FUNCTION "GestioneUscite" : VOID
TITLE =Gestione Uscite
//Gestisce le uscite controllando anche che siano rispettate le opportune
//sicurezze
VERSION : 0.1

BEGIN
NETWORK
TITLE =Uilità varie
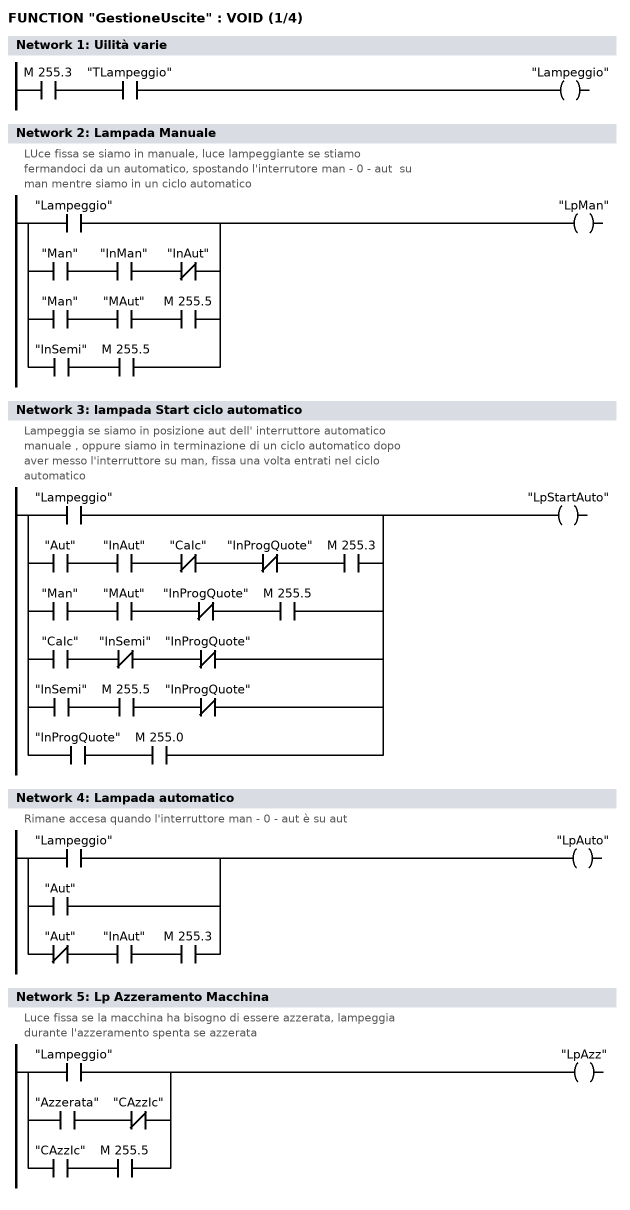
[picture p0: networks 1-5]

      U     M    255.3;
      U     "TLampeggio";
      =     "Lampeggio";


NETWORK
TITLE =Lampada Manuale
//LUce fissa se siamo in manuale, luce lampeggiante se stiamo
//fermandoci da un automatico, spostando l'interrutore man - 0 - aut  su
//man mentre siamo in un ciclo automatico
      O     "Lampeggio";
      O(    ;
      U     "Man";
      U     "InMan";
      UN    "InAut";
      )     ;
      O(    ;
      U     "Man";
      U     "MAut";
      U     M    255.5;
      )     ;
      O(    ;
      U     "InSemi";
      U     M    255.5;
      )     ;
      =     "LpMan";



NETWORK
TITLE =lampada Start ciclo automatico
//Lampeggia se siamo in posizione aut dell' interruttore automatico
//manuale , oppure siamo in terminazione di un ciclo automatico dopo
//aver messo l'interruttore su man, fissa una volta entrati nel ciclo
//automatico
      O     "Lampeggio";
      O(    ;
      U     "Aut";
      U     "InAut";
      UN    "CaIc";
      UN    "InProgQuote";
      U     M    255.3;
      )     ;
      O(    ;
      U     "Man";
      U     "MAut";
      UN    "InProgQuote";
      U     M    255.5;
      )     ;
      O(    ;
      U     "CaIc";
      UN    "InSemi";
      UN    "InProgQuote";
      )     ;
      O(    ;
      U     "InSemi";
      U     M    255.5;
      UN    "InProgQuote";
      )     ;
      O(    ;
      U     "InProgQuote";
      U     M    255.0;
      )     ;
      =     "LpStartAuto";


NETWORK
TITLE =Lampada automatico
//Rimane accesa quando l'interruttore man - 0 - aut è su aut
      O     "Lampeggio";
      O     "Aut";
      O(    ;
      UN    "Aut";
      U     "InAut";
      U     M    255.3;
      )     ;
      =     "LpAuto";


NETWORK
TITLE =Lp Azzeramento Macchina
//Luce fissa se la macchina ha bisogno di essere azzerata, lampeggia
//durante l'azzeramento spenta se azzerata

      O     "Lampeggio";
      O(    ;
      U     "Azzerata";
      UN    "CAzzIc";
      )     ;
      O(    ;
      U     "CAzzIc";
      U     M    255.5;
      )     ;
      =     "LpAzz";

NETWORK
TITLE =Lampada allarmi
//Se la macchina è in allarme, lampeggia
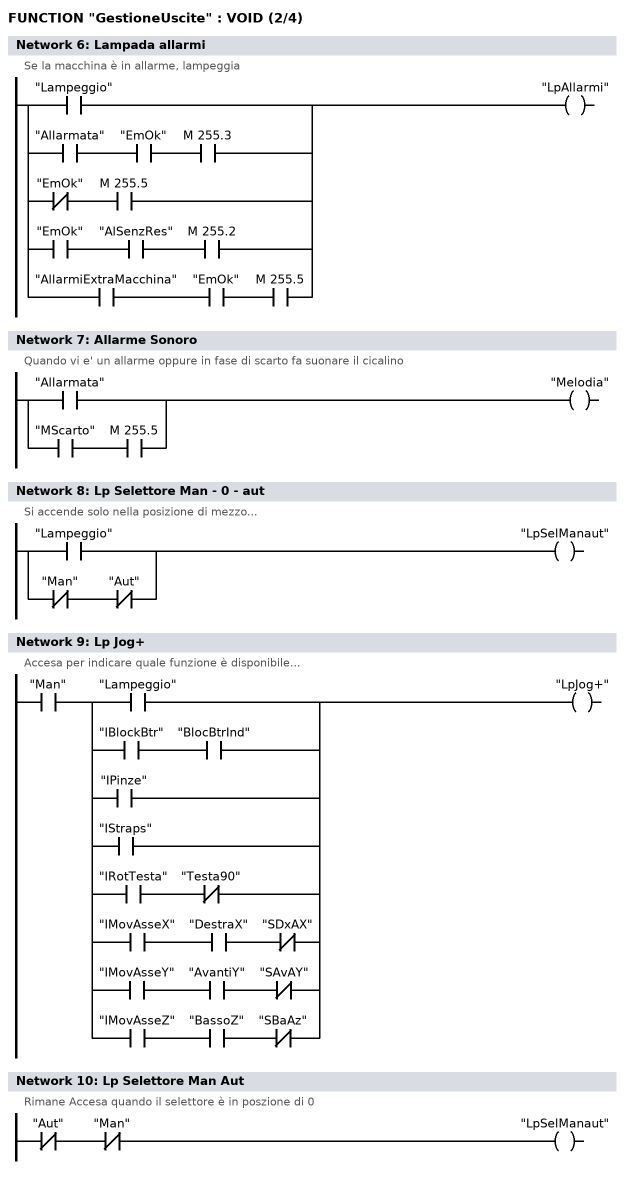
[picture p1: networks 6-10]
      O     "Lampeggio";
      O(    ;
      U     "Allarmata";
      U     "EmOk";
      U     M    255.3;
      )     ;
      O(    ;
      UN    "EmOk";
      U     M    255.5;
      )     ;
      O(    ;
      U     "EmOk";
      U     "AlSenzRes";
      U     M    255.2;
      )     ;
      O(    ;
      U     "AllarmiExtraMacchina";
      U     "EmOk";
      U     M    255.5;
      )     ;
      =     "LpAllarmi";


NETWORK
TITLE =Allarme Sonoro
//Quando vi e' un allarme oppure in fase di scarto fa suonare il cicalino
      O     "Allarmata";
      O(    ;
      U     "MScarto";
      U     M    255.5;
      )     ;
      =     "Melodia";


NETWORK
TITLE =Lp Selettore Man - 0 - aut
//Si accende solo nella posizione di mezzo...
      O     "Lampeggio";
      O(    ;
      UN    "Man";
      UN    "Aut";
      )     ;
      =     "LpSelManaut";

NETWORK
TITLE =Lp Jog+
//Accesa per indicare quale funzione è disponibile...
      U     "Man";
      U(    ;
      O     "Lampeggio";
      O(    ;
      U     "IBlockBtr";
      U     "BlocBtrInd";
      )     ;
      O     "IPinze";
      O     "IStraps";
      O(    ;
      U     "IRotTesta";
      UN    "Testa90";
      )     ;
      O(    ;
      U     "IMovAsseX";
      U     "DestraX";
      UN    "SDxAX";
      )     ;
      O(    ;
      U     "IMovAsseY";
      U     "AvantiY";
      UN    "SAvAY";
      )     ;
      O(    ;
      U     "IMovAsseZ";
      U     "BassoZ";
      UN    "SBaAz";
      )     ;
      )     ;
      =     "LpJog+";


NETWORK
TITLE =Lp Selettore Man Aut
//Rimane Accesa quando il selettore è in poszione di 0
      UN    "Aut";
      UN    "Man";
      =     "LpSelManaut";


NETWORK
TITLE =Motore pompa olio
//Fa Partire la pompa dell'olio
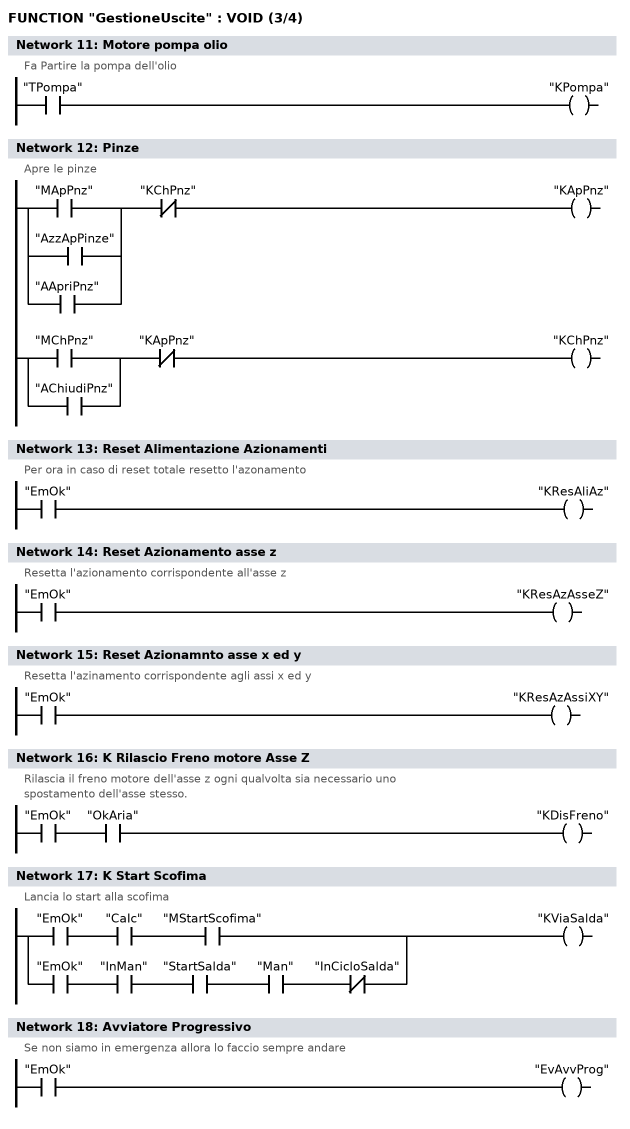
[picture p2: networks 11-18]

      U     "TPompa";
      =     "KPompa";

NETWORK
TITLE =Pinze
//Apre le pinze
      U(    ;
      O     "MApPnz";
      O     "AzzApPinze";
      O     "AApriPnz";
      )     ;
      UN    "KChPnz";
      =     "KApPnz";

      U(    ;
      O     "MChPnz";
      O     "AChiudiPnz";
      )     ;
      UN    "KApPnz";
      =     "KChPnz";


NETWORK
TITLE =Reset Alimentazione Azionamenti
//Per ora in caso di reset totale resetto l'azonamento

      U     "EmOk";
      =     "KResAliAz";

NETWORK
TITLE =Reset Azionamento asse z
//Resetta l'azionamento corrispondente all'asse z
      U     "EmOk";
      =     "KResAzAsseZ";


NETWORK
TITLE =Reset Azionamnto asse x ed y
//Resetta l'azinamento corrispondente agli assi x ed y

      U     "EmOk";
      =     "KResAzAssiXY";

NETWORK
TITLE =K Rilascio Freno motore Asse Z
//Rilascia il freno motore dell'asse z ogni qualvolta sia necessario uno
//spostamento dell'asse stesso.
      U     "EmOk";
      U     "OkAria";
      =     "KDisFreno";


NETWORK
TITLE =K Start Scofima
//Lancia lo start alla scofima
      O(    ;
      U     "EmOk";
      U     "CaIc";
      U     "MStartScofima";
      )     ;
      O(    ;
      U     "EmOk";
      U     "InMan";
      U     "StartSalda";
      U     "Man";
      UN    "InCicloSalda";
      )     ;
      =     "KViaSalda";

NETWORK
TITLE =Avviatore Progressivo
//Se non siamo in emergenza allora lo faccio sempre andare
      U     "EmOk";
      =     "EvAvvProg";


NETWORK
TITLE =Blocco BAtteria
//Manovra il bloccabatteria
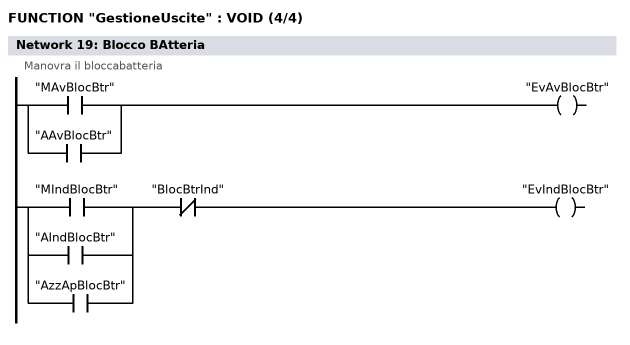
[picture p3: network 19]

      O     "MAvBlocBtr";
      O     "AAvBlocBtr";
      =     "EvAvBlocBtr";


      U(    ;
      O     "MIndBlocBtr";
      O     "AIndBlocBtr";
      O     "AzzApBlocBtr";
      )     ;
      UN    "BlocBtrInd";
      =     "EvIndBlocBtr";

NETWORK
TITLE =Rotazione testa
//Si occupa di ruotare la testa. Nota: per la rotazione, la testa deve essere
//alta, in quota sicurezza, il motore dell'asse z fermo.
      U     "DB ASSE Z".PAST1_13_MotoreFermo;
      U     "DB ASSE Z".PAST1_10_RaggPosRif;
      U(    ;
      L     "DbPosizioni".QuotaSicurezzaAsseZ;
      L     "DB ASSE Z".XRETP;
      -D    ;
      DTB   ;
      SLD   4;
      SRD   8;
      L     0;
      >=D   ;
      )     ;
      =     "OkRotTesta";

//  U     "OkRotTesta"
      UN    "Testa90";
      U(    ;
      O     "MRot90";
      O     "ARot90";
      )     ;
      =     "EvTesta90";

//      U     "OkRotTesta"
      UN    "Testa0";
      U(    ;
      O     "MRot0";
      O     "ARot0";
      )     ;
      =     "EvTesta0";


NETWORK
TITLE =Raffreddamento
//Aziona la valvola di raffreddamento
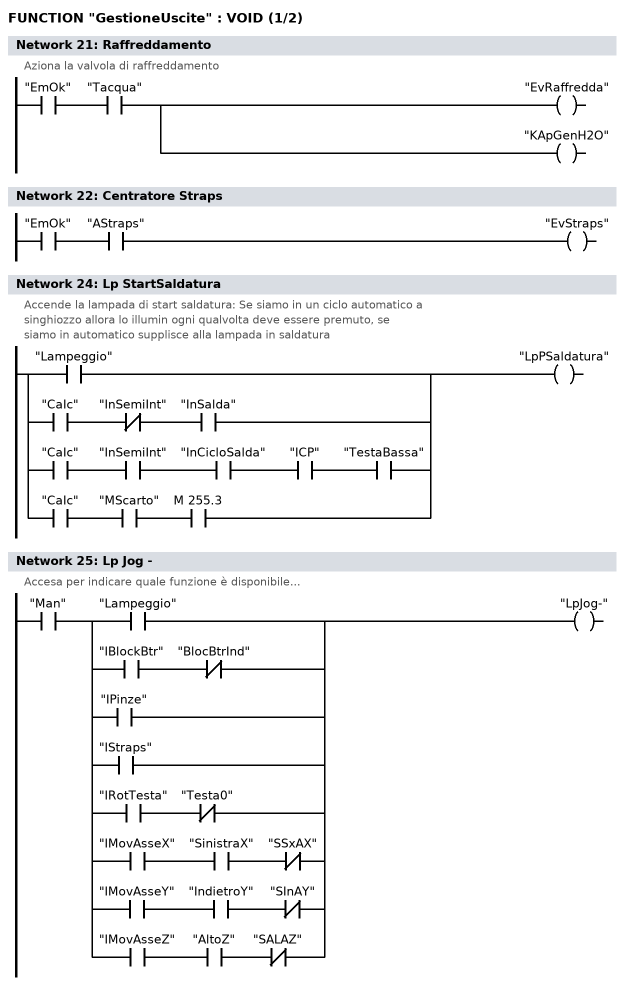
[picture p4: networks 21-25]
      U     "EmOk";
      U     "Tacqua";
      =     "EvRaffredda";
      =     "KApGenH2O";
NETWORK
TITLE =Centratore Straps

      U     "EmOk";
      U     "AStraps";
      =     "EvStraps";


NETWORK
TITLE =Espulsore (Non presente su questa macchina /Versione A)
//Gestisce il movimeto dell'espulsore
//NOTA: L'espulsore non e' presente su questa macchina, versione A della pinza
//(pinza 1)

//      U(
//     O     "MAvEspulsore"
//      O     "AAvEsp"
//      )
//      UN    "EspAv"
//      U     "BarraIndietro"
//      UN    "BarraAvanti"
//      =     "EvAvEsp"

//      U(
//      O     "MIndEspulsore"
//      O     "AIndEsp"
//      O     "AzzIndEsp"
//      )
//      UN    "EspInd"
//      =     "EvIndEsp"

NETWORK
TITLE =Lp StartSaldatura
//Accende la lampada di start saldatura: Se siamo in un ciclo automatico a
//singhiozzo allora lo illumin ogni qualvolta deve essere premuto, se
//siamo in automatico supplisce alla lampada in saldatura
      O     "Lampeggio";
      O(    ;
      U     "CaIc";
      UN    "InSemiInt";
      U     "InSalda";
      )     ;
      O(    ;
      U     "CaIc";
      U     "InSemiInt";
      U     "InCicloSalda";
      U     "ICP";
      U     "TestaBassa";
      )     ;
      O(    ;
      U     "CaIc";
      U     "MScarto";
      U     M    255.3;
      )     ;
      =     "LpPSaldatura";


NETWORK
TITLE =Lp Jog -
//Accesa per indicare quale funzione è disponibile...

      U     "Man";
      U(    ;
      O     "Lampeggio";
      O(    ;
      U     "IBlockBtr";
      UN    "BlocBtrInd";
      )     ;
      O     "IPinze";
      O     "IStraps";
      O(    ;
      U     "IRotTesta";
      UN    "Testa0";
      )     ;
      O(    ;
      U     "IMovAsseX";
      U     "SinistraX";
      UN    "SSxAX";
      )     ;
      O(    ;
      U     "IMovAsseY";
      U     "IndietroY";
      UN    "SInAY";
      )     ;
      O(    ;
      U     "IMovAsseZ";
      U     "AltoZ";
      UN    "SALAZ";
      )     ;
      )     ;
      =     "LpJog-";


NETWORK
TITLE =Segnalazioni di servizio
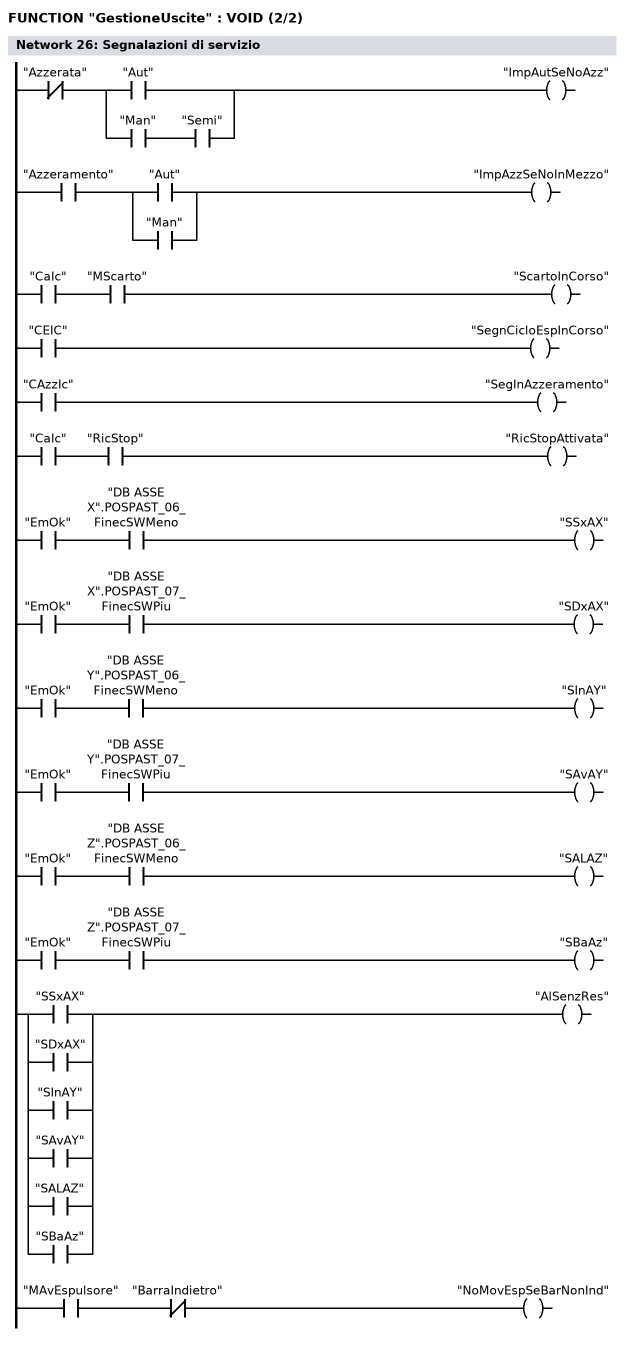
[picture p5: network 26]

      UN    "Azzerata";
      U(    ;
      O     "Aut";
      O(    ;
      U     "Man";
      U     "Semi";
      )     ;
      )     ;
      =     "ImpAutSeNoAzz";


      U     "Azzeramento";
      U(    ;
      O     "Aut";
      O     "Man";
      )     ;
      =     "ImpAzzSeNoInMezzo";


      U     "CaIc";
      U     "MScarto";
      =     "ScartoInCorso";

      U     "CEIC";
      =     "SegnCicloEspInCorso";

      U     "CAzzIc";
      =     "SegInAzzeramento";

      U     "CaIc";
      U     "RicStop";
      =     "RicStopAttivata";


//      U     "CaIc"
//      =     "RicSbloccoRipari"

// Inserire qui i bit o quello
// che si vuole controllare e magicamente
// al verificarsi delle condizioni
// inserite appare un bel messaggio
// sul pannellino.....
//      =     "IYSTMTISW"


// Controllo dei finecorsa software
// e relativa visualizzazione
// del messaggio

      U     "EmOk";
      U     "DB ASSE X".POSPAST_06_FinecSWMeno;
      =     "SSxAX";

      U     "EmOk";
      U     "DB ASSE X".POSPAST_07_FinecSWPiu;
      =     "SDxAX";

      U     "EmOk";
      U     "DB ASSE Y".POSPAST_06_FinecSWMeno;
      =     "SInAY";

      U     "EmOk";
      U     "DB ASSE Y".POSPAST_07_FinecSWPiu;
      =     "SAvAY";

      U     "EmOk";
      U     "DB ASSE Z".POSPAST_06_FinecSWMeno;
      =     "SALAZ";

      U     "EmOk";
      U     "DB ASSE Z".POSPAST_07_FinecSWPiu;
      =     "SBaAz";

      O     "SSxAX";
      O     "SDxAX";
      O     "SInAY";
      O     "SAvAY";
      O     "SALAZ";
      O     "SBaAz";
      =     "AlSenzRes";


// L' espulsore non si puo' muovere
// se la barra non e' indietro neppure
// in manuale

      U     "MAvEspulsore";
      UN    "BarraIndietro";
      =     "NoMovEspSeBarNonInd";


NETWORK
TITLE =Visualizzazione Override Attivo

// Ogni asse deve essere
// interrogato separatamente, a seconda
// di quale sia segnato sulla pulsantiera

// Se muovo l'asse X carico
// l'ovveride di X !

      U     "MMan";
      U     "IMovAsseX";
      SPB   ccx;
      SPA   nox;

ccx:  NOP   0;
      L     "DB ASSE X".OVERRIDE;
      T     "DbDati".OverrideAttivo;
      SPA   eovo;

nox:  NOP   0;

// Se muovo l'asse Y carico override di Y

      U     "MMan";
      U     "IMovAsseY";
      SPB   ccy;
      SPA   noy;

ccy:  NOP   0;
      L     "DB ASSE Y".OVERRIDE;
      T     "DbDati".OverrideAttivo;
      SPA   eovo;

noy:  NOP   0;

// Se muovo l'asse Z carico...

      U     "MMan";
      U     "IMovAsseZ";
      SPB   ccz;
      SPA   noz;

ccz:  NOP   0;
      L     "DB ASSE Z".OVERRIDE;
      T     "DbDati".OverrideAttivo;
      SPA   eovo;


// se non sono in manuale, un
// ovveride vale l'altro...

noz:  L     "DB ASSE X".OVERRIDE;
      T     "DbDati".OverrideAttivo;

eovo: NOP   0;



NETWORK
TITLE =Segnalazione scarto avvenuto da DIVE

      U     "diveReject_Signal";
      U     M    255.3;
      =     "diveReject_Lamp_";



END_FUNCTION

